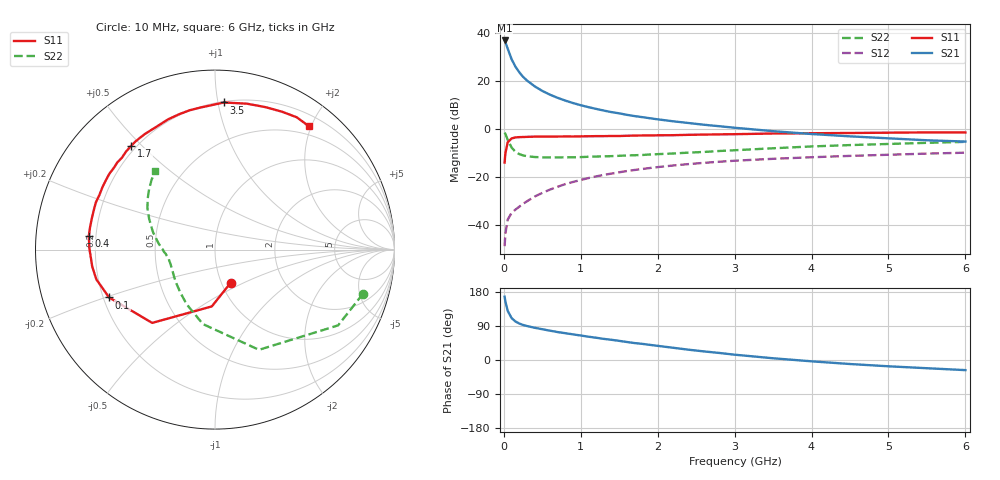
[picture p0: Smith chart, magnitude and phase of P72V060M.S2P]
! SIEMENS Small Signal Semiconductors
! BFP196
! Si NPN RF Bipolar Junction Transistor in SOT143
! VCE = 2 V  IC = 60 mA
! Common Emitter S-Parameters:  May  1996
# GHz  S  MA  R  50
!  f  S11  S21  S12  S22
! GHz  MAG  ANG  MAG  ANG  MAG  ANG  MAG  ANG
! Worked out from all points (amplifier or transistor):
!   36 points, 10 MHz to 6 GHz, reference 50 ohm
!   highest |S21| = 37.1 dB at 10 MHz (marker M1)
!   |S21| within 3 dB of that: start of sweep to 45.45 MHz
!   unconditionally stable (mu >= 1): 391 MHz to 4.744 GHz
!   at 250 MHz: K = 0.90, MSG = 26.5 dB, |S12| = -31.0 dB
!   at 1.4 GHz: K = 1.09, MAG = 10.9 dB, |S12| = -18.4 dB
!   at 6 GHz: K = 0.99, MSG = 2.3 dB, |S12| = -9.7 dB
!   S11 on the Smith chart (normalised r, x): 10 MHz: 1.10, -0.43; 100 MHz: 0.22, -0.21; 400 MHz: 0.17, +0.05; 1.7 GHz: 0.18, +0.47; 3.5 GHz: 0.21, +1.04; 6 GHz: 0.36, +1.97
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0.01  0.2047 -64.8  71.22 167.1  0.0037 78.7  0.8605 -16.6
0.02  0.317 -93.2  65.97 154.5  0.0068 68.9  0.8055 -31.6
0.05  0.5379 -130.6  48.06 129.9  0.0132 53.3  0.6098 -66.3
0.1  0.6476 -155.7  29.15 110.8  0.0182 49.6  0.4204 -99.2
0.15  0.6815 -165.9  20.37 101.8  0.0213 51.2  0.3429 -117.5
0.2  0.6905 -172.1  15.55 96.3  0.0245 55.0  0.3065 -129.3
0.25  0.6939 -176.9  12.46 92.5  0.0282 56.5  0.2871 -138.2
0.3  0.6992 179.9  10.45 89.7  0.0318 59.9  0.2774 -144.0
0.4  0.707 174.0  7.914 85.1  0.0399 62.4  0.266 -152.4
0.5  0.7072 170.0  6.333 81.2  0.0476 63.6  0.262 -158.0
0.6  0.7081 165.6  5.284 77.4  0.0558 64.3  0.2607 -161.6
0.7  0.7105 161.6  4.545 73.7  0.064 64.2  0.2613 -164.5
0.9  0.7123 154.7  3.536 67.6  0.0805 62.9  0.2629 -168.9
1.1  0.7199 148.0  2.909 61.5  0.097 61.1  0.2692 -171.8
1.3  0.7246 141.1  2.468 55.7  0.113 58.3  0.2746 -174.7
1.7  0.7434 128.9  1.894 44.7  0.1429 52.9  0.2899 -179.9
2.2  0.7579 115.6  1.476 32.3  0.1772 45.3  0.315 174.0
2.8  0.7887 100.5  1.166 18.6  0.2123 36.3  0.3553 165.0
3.5  0.8213 86.5  0.919 4.6  0.2442 26.2  0.4048 155.0
4.5  0.8423 70.4  0.717 -10.6  0.281 14.2  0.4717 142.6
5.5  0.8666 58.3  0.594 -21.7  0.3132 3.4  0.5252 132.3
6  0.8638 52.7  0.558 -26.7  0.3275 -2.4  0.55 127.3
